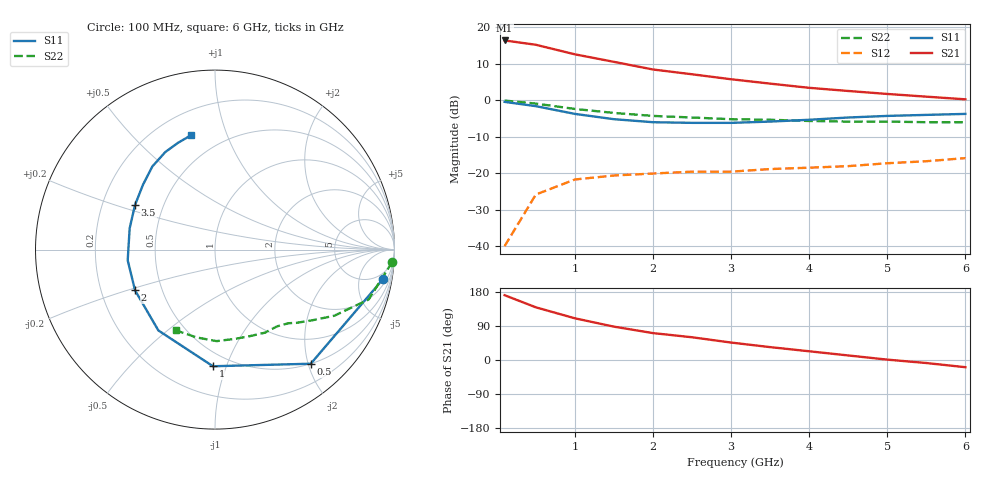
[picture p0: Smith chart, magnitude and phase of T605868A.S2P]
!AT-60586
!S-PARAMETERS at Vce=8V  Ic=2mA.  LAST UPDATED 07-21-92
# ghz s ma r 50
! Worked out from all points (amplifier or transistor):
!   13 points, 100 MHz to 6 GHz, reference 50 ohm
!   highest |S21| = 16.4 dB at 100 MHz (marker M1)
!   |S21| within 3 dB of that: start of sweep to 846.8 MHz
!   unconditionally stable (mu >= 1): 2.516 GHz to end of sweep
!   at 1 GHz: K = 0.50, MSG = 17.2 dB, |S12| = -21.7 dB
!   at 3 GHz: K = 1.19, MAG = 10.0 dB, |S12| = -19.6 dB
!   at 6 GHz: K = 1.09, MAG = 6.2 dB, |S12| = -15.9 dB
!   S11 on the Smith chart (normalised r, x): 100 MHz: 3, -11; 500 MHz: 0.50, -2.04; 1 GHz: 0.40, -0.90; 2 GHz: 0.35, -0.21; 3.5 GHz: 0.34, +0.23; 6 GHz: 0.34, +0.75
0.1  0.95 -10.0  6.6 171.0  0.01 82.0  0.99 -4.0
0.5  0.83 -50.0  5.76 139.0  0.051 61.0  0.9 -18.0
1  0.65 -91.0  4.26 110.0  0.082 43.0  0.76 -29.0
1.5  0.55 -125.0  3.36 88.0  0.093 36.0  0.67 -36.0
2  0.5 -153.0  2.64 71.0  0.099 30.0  0.61 -42.0
2.5  0.49 -173.0  2.27 60.0  0.105 32.0  0.58 -45.0
3  0.49 166.0  1.94 46.0  0.105 32.0  0.55 -51.0
3.5  0.51 151.0  1.69 34.0  0.114 28.0  0.54 -59.0
4  0.54 138.0  1.48 23.0  0.119 30.0  0.52 -68.0
4.5  0.58 127.0  1.34 12.0  0.125 30.0  0.51 -77.0
5  0.61 117.0  1.22 1.0  0.137 30.0  0.51 -89.0
5.5  0.63 109.0  1.12 -8.0  0.146 30.0  0.5 -102.0
6  0.65 102.0  1.03 -19.0  0.161 28.0  0.5 -116.0
